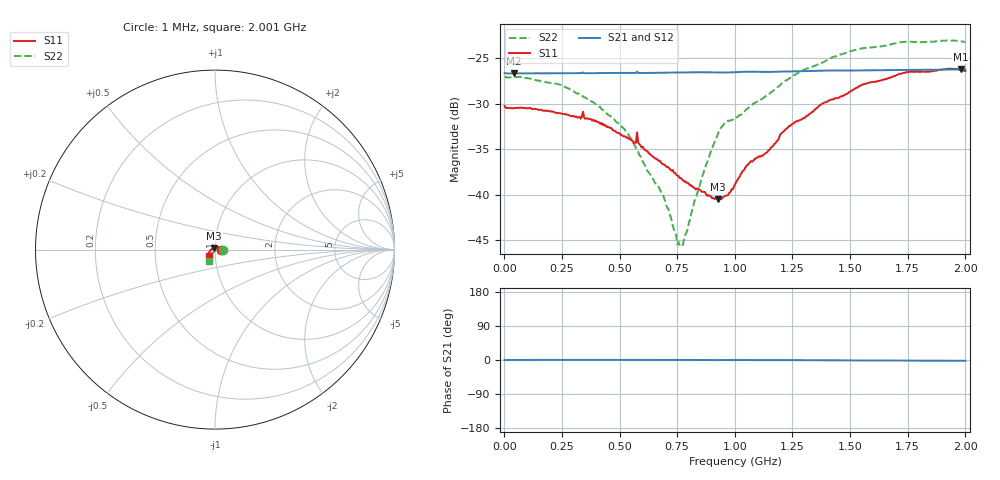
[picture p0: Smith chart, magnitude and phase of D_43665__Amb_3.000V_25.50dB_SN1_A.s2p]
! device id: 43665_
! dir: \\malibu\benchdata\1_engineers\tn_data\43665_75ohm\new\sparar\43665_\amb\3p000v\25p50db
! Serial: 1
! Insertion: A
! Temp: Amb
! VDD: 3.000V
! Attenuation Step: 25.50dB
! IDD: 1.449013e+00mA
! FILE NAME
! DATE 03-27-2009 08:39:38
! CORRECTED  DATA
#  Hz  S  RI  R  75
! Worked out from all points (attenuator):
!   401 points, 1 MHz to 2.001 GHz, reference 75 ohm
!   highest |S21| = -26.21 dB at 1.981 GHz (marker M1); lowest = -26.7 dB at 41 MHz (marker M2)
!   lowest |S11| = -40.5 dB at 926 MHz (marker M3), VSWR 1.02, Z = 74.3 + j1.2 ohm
!   |S11| at or under -10 dB: start of sweep to end of sweep
!   |S22| runs from -45.7 to -23.0 dB; largest |S21 - S12| = 0.00073
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1000000  0.0307 -0.000374  0.0467 -6.22e-05  0.0468 -9.18e-05  0.0445 -0.000493
4.1e7  0.0298 0.00107  0.0465 5.49e-05  0.0465 1.91e-05  0.0444 0.00069
2.36e8  0.0275 0.00611  0.0466 0.000284  0.0466 0.000175  0.0401 0.00552
3.36e8  0.0255 0.00806  0.0467 0.000349  0.0467 0.000231  0.0344 0.00668
5.21e8  0.0177 0.0111  0.0468 0.000177  0.0468 0.000228  0.0225 0.0042
5.81e8  0.0152 0.0118  0.0468 0.00013  0.0468 0.000187  0.0168 0.00353
6.71e8  0.00998 0.0116  0.0469 0.00024  0.0469 0.000316  0.0109 -0.000264
7.01e8  0.00845 0.0115  0.047 0.000236  0.047 0.000338  0.0089 -0.00116
7.56e8  0.00558 0.0114  0.0471 0.000172  0.0471 0.000257  0.00409 -0.00366
7.71e8  0.00492 0.0111  0.0471 0.000144  0.0471 0.000247  0.00261 -0.00449
8.66e8  -0.000852 0.0103  0.0472 -2.09e-05  0.0472 0.000117  -0.00439 -0.0127
9.26e8  -0.00487 0.00808  0.0471 -0.00016  0.0472 3.02e-05  -0.0111 -0.0183
9.61e8  -0.00654 0.00738  0.0471 -1.31e-05  0.0471 0.000177  -0.0165 -0.0185
1.001e9  -0.00887 0.00712  0.0472 0.000113  0.0473 0.000302  -0.0192 -0.0178
1.061e9  -0.0138 0.00556  0.0475 -0.0001  0.0476 0.000111  -0.0207 -0.0219
1.141e9  -0.0169 0.00245  0.0474 -0.000245  0.0475 -3.28e-05  -0.0226 -0.027
1.226e9  -0.0231 -0.00148  0.0476 -0.000241  0.0478 -1.72e-05  -0.0263 -0.0336
1.336e9  -0.0277 -0.00679  0.048 -0.000368  0.0482 -0.000163  -0.0298 -0.041
1.546e9  -0.0354 -0.0183  0.0483 -0.00101  0.0485 -0.000824  -0.0339 -0.054
1.671e9  -0.0367 -0.0243  0.0485 -0.00123  0.0486 -0.0011  -0.0346 -0.0572
1.981e9  -0.0333 -0.0357  0.0489 -0.00179  0.0491 -0.00173  -0.0331 -0.0616
2.001e9  -0.0324 -0.0353  0.0489 -0.00176  0.049 -0.00179  -0.0329 -0.0608
